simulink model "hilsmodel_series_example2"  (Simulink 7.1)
settings: Solver=ode3  StartTime=0.0  StopTime=1800  FixedStep=hilsmdl.simulation.stepsize.value  MaxStep=0.01  RelTol=1e-3  AbsTol=1e-3
undefined symbols (not defined in the file or in its folder): hilsmdl
libraries: HILS_model_library x9, simulink_extras x1

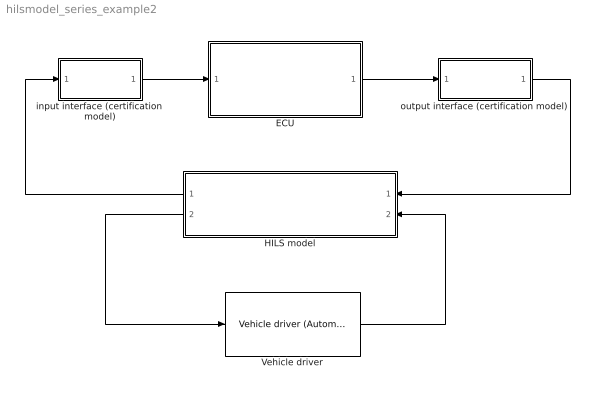
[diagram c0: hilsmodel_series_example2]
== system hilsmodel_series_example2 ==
  ECU : Subsystem  mask{dat=hilsmdl.ecu}
      mask prompts: dat "Data set for ECU"
  HILS model : Subsystem  Orientation=left
  Vehicle driver : HILS_model_library/Driver/Vehicle driver (Automatic)  dat=hilsmdl.driverautomatic
  input interface (certification model) : Subsystem
  output interface (certification model) : Subsystem
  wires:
  input interface (certification model)/1(to ECU) -> ECU/1(sensor in)
  ECU/1(cmd out) -> output interface (certification model)/1(from ECU)
  HILS model/1(To Ctrl) -> input interface (certification model)/1(plant in)
  output interface (certification model)/1(cmd out) -> HILS model/1(From Ctrl)
  Vehicle driver/1 -> HILS model/2(From driver)
  HILS model/2(To driver) -> Vehicle driver/1

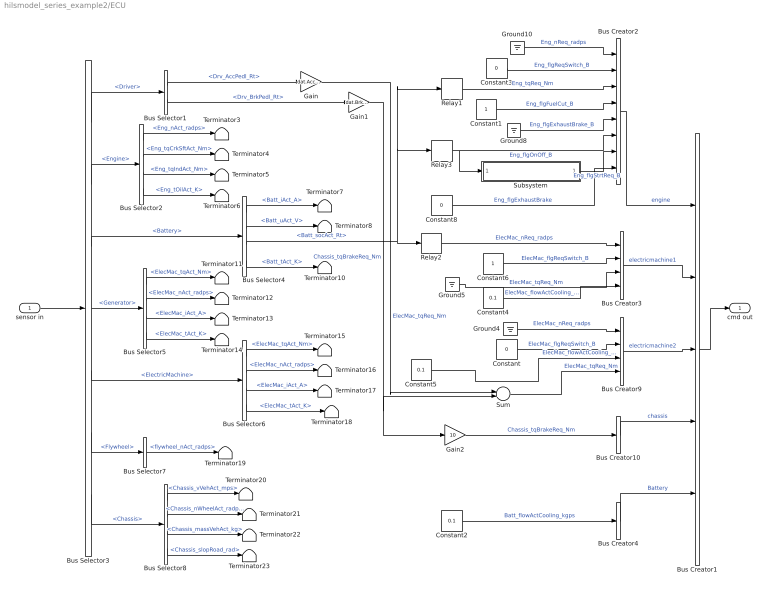
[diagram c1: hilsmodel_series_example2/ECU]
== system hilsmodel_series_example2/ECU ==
  sensor in : Inport
  Bus Creator1 : BusCreator  Inputs=5
  Bus Creator10 : BusCreator  Inputs=1
  Bus Creator2 : BusCreator  Inputs=8
  Bus Creator3 : BusCreator
  Bus Creator4 : BusCreator  Inputs=1
  Bus Creator9 : BusCreator
  Bus Selector1 : BusSelector  OutputSignals=Drv_AccPedl_Rt,Drv_BrkPedl_Rt
  Bus Selector2 : BusSelector  OutputSignals=Eng_nAct_radps,Eng_tqCrkSftAct_Nm,Eng_tqIndAct_Nm,Eng_tOilAct_K
  Bus Selector3 : BusSelector  OutputSignals=Driver,Engine,Battery,Generator,ElectricMachine,Flywheel,Chassis
  Bus Selector4 : BusSelector  OutputSignals=Batt_iAct_A,Batt_uAct_V,Batt_socAct_Rt,Batt_tAct_K
  Bus Selector5 : BusSelector  OutputSignals=ElecMac_tqAct_Nm,ElecMac_nAct_radps,ElecMac_iAct_A,ElecMac_tAct_K
  Bus Selector6 : BusSelector  OutputSignals=ElecMac_tqAct_Nm,ElecMac_nAct_radps,ElecMac_iAct_A,ElecMac_tAct_K
  Bus Selector7 : BusSelector  OutputSignals=flywheel_nAct_radps
  Bus Selector8 : BusSelector  OutputSignals=Chassis_vVehAct_mps,Chassis_nWheelAct_radps,Chassis_massVehAct_kg,Chassis_slopRoad_rad
  Constant : Constant  Value=0
  Constant1 : Constant
  Constant2 : Constant  Value=0.1
  Constant3 : Constant  Value=0
  Constant4 : Constant  Value=0.1
  Constant5 : Constant  Value=0.1
  Constant6 : Constant
  Constant8 : Constant  Value=0
  Gain : Gain  Gain=dat.AccPedalGain.value
  Gain1 : Gain  Gain=dat.BrkPedalGain.value
  Gain2 : Gain  Gain=10
  Ground{4..5,8,10} (4 alike) : Ground
  Relay1 : Relay  OnSwitchValue=dat.socstrategy.EngineOff.value  OffSwitchValue=dat.socstrategy.EngineOn.value  OnOutputValue=0  OffOutputValue=dat.socstrategy.torqueref.value
  Relay2 : Relay  OnSwitchValue=dat.socstrategy.EngineOff.value  OffSwitchValue=dat.socstrategy.EngineOn.value  OnOutputValue=0  OffOutputValue=dat.socstrategy.speedref.value
  Relay3 : Relay  OnSwitchValue=dat.socstrategy.EngineOff.value  OffSwitchValue=dat.socstrategy.EngineOn.value  OnOutputValue=0  OffOutputValue=1
  Subsystem : Subsystem
  Sum : Sum  Inputs=|+-
  Terminator{3..8,10..23} (20 alike) : Terminator
  cmd out : Outport
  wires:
  Bus Creator10/1 -> Bus Creator1/4  "chassis"
  Constant/1 -> Bus Creator9/2  "ElecMac_flgReqSwitch_B"
  Ground4/1 -> Bus Creator9/1  "ElecMac_nReq_radps"
  Bus Creator1/1 -> cmd out/1
  Bus Creator2/1 -> Bus Creator1/1  "engine"
  Ground10/1 -> Bus Creator2/1  "Eng_nReq_radps"
  Constant3/1 -> Bus Creator2/2  "Eng_flgReqSwitch_B"
  Bus Creator3/1 -> Bus Creator1/2  "electricmachine1"
  Constant6/1 -> Bus Creator3/2  "ElecMac_flgReqSwitch_B"
  Ground5/1 -> Bus Creator3/3  "ElecMac_tqReq_Nm"
  Bus Creator9/1 -> Bus Creator1/3  "electricmachine2"
  Bus Selector3/4 -> Bus Selector5/1  "<Generator>"
  sensor in/1 -> Bus Selector3/1
  Bus Selector3/1 -> Bus Selector1/1  "<Driver>"
  Bus Selector3/2 -> Bus Selector2/1  "<Engine>"
  Bus Selector3/3 -> Bus Selector4/1  "<Battery>"
  Bus Selector3/5 -> Bus Selector6/1  "<ElectricMachine>"
  Bus Selector3/6 -> Bus Selector7/1  "<Flywheel>"
  Bus Selector3/7 -> Bus Selector8/1  "<Chassis>"
  Bus Selector1/1 -> Gain/1  "<Drv_AccPedl_Rt>"
  Bus Selector1/2 -> Gain1/1  "<Drv_BrkPedl_Rt>"
  Bus Selector2/1 -> Terminator3/1  "<Eng_nAct_radps>"
  Bus Selector2/2 -> Terminator4/1  "<Eng_tqCrkSftAct_Nm>"
  Bus Selector2/3 -> Terminator5/1  "<Eng_tqIndAct_Nm>"
  Bus Selector2/4 -> Terminator6/1  "<Eng_tOilAct_K>"
  Bus Selector4/1 -> Terminator7/1  "<Batt_iAct_A>"
  Bus Selector4/2 -> Terminator8/1  "<Batt_uAct_V>"
  Bus Selector4/3 -> Relay2/1, Relay1/1, Relay3/1  "<Batt_socAct_Rt>"
  Bus Selector4/4 -> Terminator10/1  "<Batt_tAct_K>"
  Bus Selector5/1 -> Terminator11/1  "<ElecMac_tqAct_Nm>"
  Bus Selector5/2 -> Terminator12/1  "<ElecMac_nAct_radps>"
  Bus Selector5/3 -> Terminator13/1  "<ElecMac_iAct_A>"
  Bus Selector5/4 -> Terminator14/1  "<ElecMac_tAct_K>"
  Bus Selector6/1 -> Terminator15/1  "<ElecMac_tqAct_Nm>"
  Bus Selector6/2 -> Terminator16/1  "<ElecMac_nAct_radps>"
  Bus Selector6/3 -> Terminator17/1  "<ElecMac_iAct_A>"
  Bus Selector6/4 -> Terminator18/1  "<ElecMac_tAct_K>"
  Bus Selector7/1 -> Terminator19/1  "<flywheel_nAct_radps>"
  Bus Selector8/1 -> Terminator20/1  "<Chassis_vVehAct_mps>"
  Bus Selector8/2 -> Terminator21/1  "<Chassis_nWheelAct_radps>"
  Bus Selector8/3 -> Terminator22/1  "<Chassis_massVehAct_kg>"
  Bus Selector8/4 -> Terminator23/1  "<Chassis_slopRoad_rad>"
  Gain/1 -> Sum/1  "ElecMac_tqReq_Nm"
  Sum/1 -> Bus Creator9/4  "ElecMac_tqReq_Nm"
  Gain1/1 -> Gain2/1, Sum/2  "Chassis_tqBrakeReq_Nm"
  Relay1/1 -> Bus Creator2/3  "Eng_tqReq_Nm"
  Relay2/1 -> Bus Creator3/1  "ElecMac_nReq_radps"
  Ground8/1 -> Bus Creator2/5  "Eng_flgExhaustBrake_B"
  Constant1/1 -> Bus Creator2/4  "Eng_flgFuelCut_B"
  Relay3/1 -> Bus Creator2/6, Subsystem/1(Engine onoff)  "Eng_flgOnOff_B"
  Subsystem/1(Starter motor ctrl) -> Bus Creator2/7  "Eng_flgStrtReq_B"
  Bus Creator4/1 -> Bus Creator1/5  "Battery"
  Constant2/1 -> Bus Creator4/1  "Batt_flowActCooling_kgps"
  Constant4/1 -> Bus Creator3/4  "ElecMac_flowActCooling_kgps"
  Constant5/1 -> Bus Creator9/3  "ElecMac_flowActCooling_kgps"
  Constant8/1 -> Bus Creator2/8  "Eng_flgExhaustBrake"
  Gain2/1 -> Bus Creator10/1  "Chassis_tqBrakeReq_Nm"

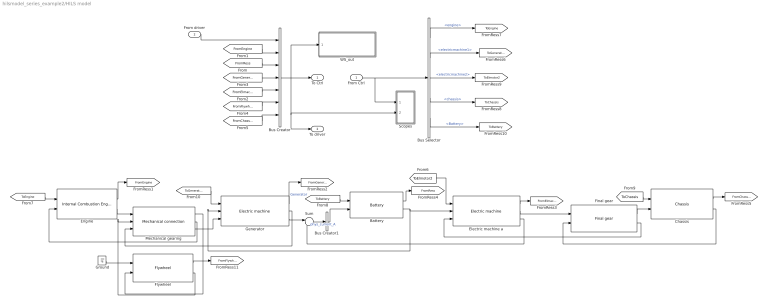
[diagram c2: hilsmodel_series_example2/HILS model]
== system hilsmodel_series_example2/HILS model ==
  From Ctrl : Inport
  From driver : Inport  Port=2
  Battery : HILS_model_library/Rechargable energy storage systems/Battery  dat=hilsmdl.battery
  Bus Creator : BusCreator  Inputs=7
  Bus Creator1 : BusCreator  Inputs=1
  Bus Selector : BusSelector  OutputSignals=engine,electricmachine1,electricmachine2,chassis,Battery
  Chassis : HILS_model_library/Chassis/Chassis  dat=hilsmdl.chassis
  Electric machine a : HILS_model_library/Energy converters/Electric machine  dat=hilsmdl.elmachinea
  Engine : HILS_model_library/Energy converters/Internal Combustion Engine  dat=hilsmdl.eng
  Final gear : HILS_model_library/Mechanical components/Final gear  dat=hilsmdl.finalgear
  Flywheel : HILS_model_library/Rechargable energy storage systems/Flywheel  dat=hilsmdl.flywheel
  Generator : HILS_model_library/Energy converters/Electric machine  dat=hilsmdl.elmachineb
  Ground : Ground
  Mechanical gearing : HILS_model_library/Mechanical components/Mechanical connection  dat=hilsmdl.mechconnection
  Scopes : Subsystem
  Sum : Sum  Inputs=|++
  WS_out : Subsystem
  To Ctrl : Outport
  To driver : Outport  Port=2
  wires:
  Bus Creator/1 -> To Ctrl/1, WS_out/1(from model), Scopes/2(plnt in), To driver/1
  From driver/1 -> Bus Creator/1
  Chassis/1 -> [FromChassis]
  From Ctrl/1 -> Scopes/1(ctrl in), Bus Selector/1
  [FromRess] -> Bus Creator/3
  Engine/1 -> [FromEngine]
  [FromEngine] -> Bus Creator/2
  [FromElmachine2] -> Bus Creator/5
  [FromGenerator1] -> Bus Creator/4
  [FromFlywheel] -> Bus Creator/6
  [FromChassis] -> Bus Creator/7
  Bus Selector/1 -> [ToEngine]  "<engine>"
  Bus Selector/2 -> [ToGenerator1]  "<electricmachine1>"
  [ToEngine] -> Engine/1
  [ToChassis] -> Chassis/1
  Electric machine a/1 -> [FromElmachine2]
  [ToElmotor2] -> Electric machine a/1
  Electric machine a/3 -> Sum/2
  Battery/2 -> Electric machine a/2, Generator/2
  Battery/1 -> [FromRess]
  [ToBattery] -> Battery/1
  Mechanical gearing/1 -> Flywheel/2
  Generator/2 -> Mechanical gearing/3
  Mechanical gearing/2 -> Engine/2
  Mechanical gearing/3 -> Generator/3
  Generator/1 -> [FromGenerator1]  "Generator"
  [ToGenerator1] -> Generator/1
  Flywheel/2 -> Mechanical gearing/2
  Flywheel/1 -> [FromFlywheel]
  Ground/1 -> Flywheel/1
  Bus Selector/4 -> [ToChassis]  "<chassis>"
  Bus Selector/3 -> [ToElmotor2]  "<electricmachine2>"
  Sum/1 -> Bus Creator1/1  "phys_current_A"
  Bus Creator1/1 -> Battery/2
  Engine/2 -> Mechanical gearing/1
  Generator/3 -> Sum/1
  Electric machine a/2 -> Final gear/1
  Final gear/2 -> Electric machine a/3
  Final gear/1 -> Chassis/2
  Chassis/2 -> Final gear/2
  Bus Selector/5 -> [ToBattery]  "<Battery>"

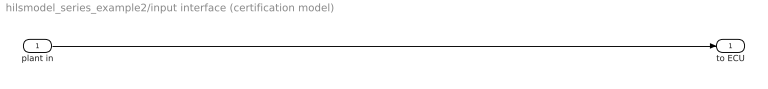
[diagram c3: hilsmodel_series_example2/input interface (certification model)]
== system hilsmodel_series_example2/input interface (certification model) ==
  plant in : Inport
  to ECU : Outport
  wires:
  plant in/1 -> to ECU/1

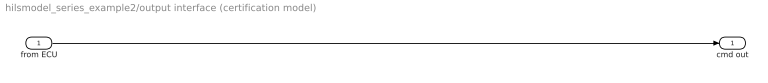
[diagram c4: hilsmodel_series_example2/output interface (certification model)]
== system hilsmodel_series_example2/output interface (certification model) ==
  from ECU : Inport
  cmd out : Outport
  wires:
  from ECU/1 -> cmd out/1

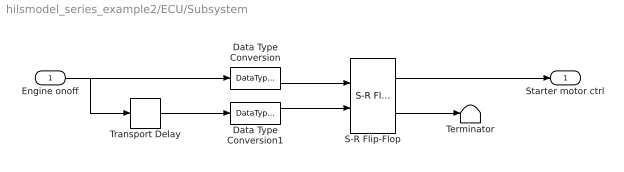
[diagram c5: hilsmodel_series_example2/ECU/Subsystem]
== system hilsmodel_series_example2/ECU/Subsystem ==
  Engine onoff : Inport
  Data Type Conversion : DataTypeConversion
  Data Type Conversion1 : DataTypeConversion
  S-R Flip-Flop : simulink_extras/Flip Flops/S-R Flip-Flop  initial_condition=0
  Terminator : Terminator
  Transport Delay : TransportDelay  DelayTime=dat.crankingtime.value
  Starter motor ctrl : Outport
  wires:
  Engine onoff/1 -> Transport Delay/1, Data Type Conversion/1
  S-R Flip-Flop/1 -> Starter motor ctrl/1
  S-R Flip-Flop/2 -> Terminator/1
  Transport Delay/1 -> Data Type Conversion1/1
  Data Type Conversion/1 -> S-R Flip-Flop/1
  Data Type Conversion1/1 -> S-R Flip-Flop/2

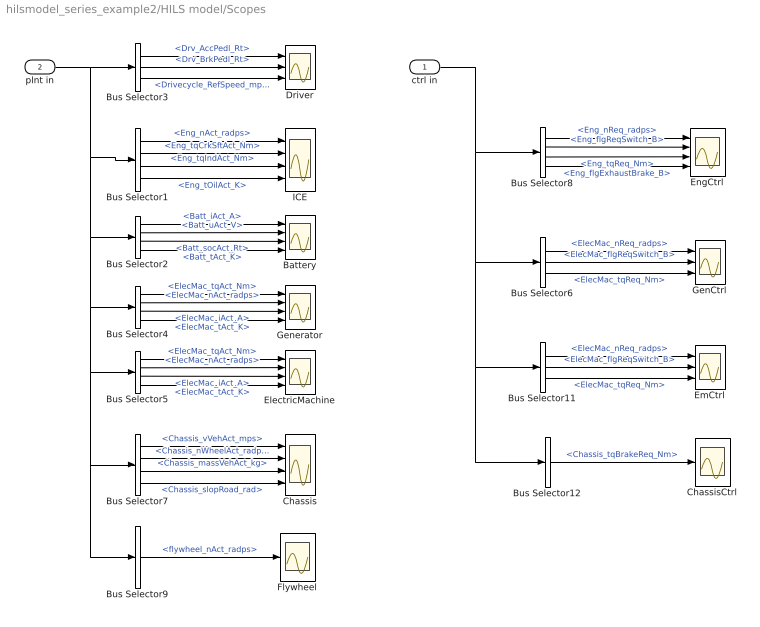
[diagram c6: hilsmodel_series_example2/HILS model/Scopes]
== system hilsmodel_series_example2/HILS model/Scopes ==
  ctrl in : Inport
  plnt in : Inport  Port=2
  Battery : Scope  NumInputPorts=4
  Bus Selector1 : BusSelector  OutputSignals=Engine.Eng_nAct_radps,Engine.Eng_tqCrkSftAct_Nm,Engine.Eng_tqIndAct_Nm,Engine.Eng_tOilAct_K
  Bus Selector11 : BusSelector  OutputSignals=electricmachine2.ElecMac_nReq_radps,electricmachine2.ElecMac_flgReqSwitch_B,electricmachine2.ElecMac_tqReq_Nm
  Bus Selector12 : BusSelector  OutputSignals=chassis.Chassis_tqBrakeReq_Nm
  Bus Selector2 : BusSelector  OutputSignals=Battery.Batt_iAct_A,Battery.Batt_uAct_V,Battery.Batt_socAct_Rt,Battery.Batt_tAct_K
  Bus Selector3 : BusSelector  OutputSignals=Driver.Drv_AccPedl_Rt,Driver.Drv_BrkPedl_Rt,Driver.Drivecycle_RefSpeed_mps
  Bus Selector4 : BusSelector  OutputSignals=Generator.ElecMac_tqAct_Nm,Generator.ElecMac_nAct_radps,Generator.ElecMac_iAct_A,Generator.ElecMac_tAct_K
  Bus Selector5 : BusSelector  OutputSignals=ElectricMachine.ElecMac_tqAct_Nm,ElectricMachine.ElecMac_nAct_radps,ElectricMachine.ElecMac_iAct_A,ElectricMachine.ElecMac_tAct_K
  Bus Selector6 : BusSelector  OutputSignals=electricmachine1.ElecMac_nReq_radps,electricmachine1.ElecMac_flgReqSwitch_B,electricmachine1.ElecMac_tqReq_Nm
  Bus Selector7 : BusSelector  OutputSignals=Chassis.Chassis_vVehAct_mps,Chassis.Chassis_nWheelAct_radps,Chassis.Chassis_massVehAct_kg,Chassis.Chassis_slopRoad_rad
  Bus Selector8 : BusSelector  OutputSignals=engine.Eng_nReq_radps,engine.Eng_flgReqSwitch_B,engine.Eng_tqReq_Nm,engine.Eng_flgExhaustBrake_B
  Bus Selector9 : BusSelector  OutputSignals=Flywheel.flywheel_nAct_radps
  Chassis : Scope  NumInputPorts=4
  ChassisCtrl : Scope
  Driver : Scope  NumInputPorts=3
  ElectricMachine : Scope  NumInputPorts=4
  EmCtrl : Scope  NumInputPorts=3
  EngCtrl : Scope  NumInputPorts=4
  Flywheel : Scope
  GenCtrl : Scope  NumInputPorts=3
  Generator : Scope  NumInputPorts=4
  ICE : Scope  NumInputPorts=4
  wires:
  Bus Selector3/1 -> Driver/1  "<Drv_AccPedl_Rt>"
  Bus Selector3/3 -> Driver/3  "<Drivecycle_RefSpeed_mps>"
  Bus Selector3/2 -> Driver/2  "<Drv_BrkPedl_Rt>"
  plnt in/1 -> Bus Selector3/1, Bus Selector1/1, Bus Selector2/1, Bus Selector5/1, Bus Selector7/1, Bus Selector9/1, Bus Selector4/1
  Bus Selector1/1 -> ICE/1  "<Eng_nAct_radps>"
  Bus Selector1/2 -> ICE/2  "<Eng_tqCrkSftAct_Nm>"
  Bus Selector1/3 -> ICE/3  "<Eng_tqIndAct_Nm>"
  Bus Selector2/1 -> Battery/1  "<Batt_iAct_A>"
  Bus Selector2/2 -> Battery/2  "<Batt_uAct_V>"
  Bus Selector2/3 -> Battery/3  "<Batt_socAct_Rt>"
  Bus Selector5/1 -> ElectricMachine/1  "<ElecMac_tqAct_Nm>"
  Bus Selector5/2 -> ElectricMachine/2  "<ElecMac_nAct_radps>"
  Bus Selector7/1 -> Chassis/1  "<Chassis_vVehAct_mps>"
  Bus Selector7/2 -> Chassis/2  "<Chassis_nWheelAct_radps>"
  Bus Selector7/3 -> Chassis/3  "<Chassis_massVehAct_kg>"
  Bus Selector7/4 -> Chassis/4  "<Chassis_slopRoad_rad>"
  ctrl in/1 -> Bus Selector8/1, Bus Selector11/1, Bus Selector12/1, Bus Selector6/1
  Bus Selector8/1 -> EngCtrl/1  "<Eng_nReq_radps>"
  Bus Selector8/2 -> EngCtrl/2  "<Eng_flgReqSwitch_B>"
  Bus Selector11/1 -> EmCtrl/1  "<ElecMac_nReq_radps>"
  Bus Selector11/2 -> EmCtrl/2  "<ElecMac_flgReqSwitch_B>"
  Bus Selector11/3 -> EmCtrl/3  "<ElecMac_tqReq_Nm>"
  Bus Selector12/1 -> ChassisCtrl/1  "<Chassis_tqBrakeReq_Nm>"
  Bus Selector1/4 -> ICE/4  "<Eng_tOilAct_K>"
  Bus Selector2/4 -> Battery/4  "<Batt_tAct_K>"
  Bus Selector4/1 -> Generator/1  "<ElecMac_tqAct_Nm>"
  Bus Selector4/2 -> Generator/2  "<ElecMac_nAct_radps>"
  Bus Selector4/3 -> Generator/3  "<ElecMac_iAct_A>"
  Bus Selector4/4 -> Generator/4  "<ElecMac_tAct_K>"
  Bus Selector5/3 -> ElectricMachine/3  "<ElecMac_iAct_A>"
  Bus Selector5/4 -> ElectricMachine/4  "<ElecMac_tAct_K>"
  Bus Selector8/3 -> EngCtrl/3  "<Eng_tqReq_Nm>"
  Bus Selector8/4 -> EngCtrl/4  "<Eng_flgExhaustBrake_B>"
  Bus Selector6/1 -> GenCtrl/1  "<ElecMac_nReq_radps>"
  Bus Selector6/2 -> GenCtrl/2  "<ElecMac_flgReqSwitch_B>"
  Bus Selector6/3 -> GenCtrl/3  "<ElecMac_tqReq_Nm>"
  Bus Selector9/1 -> Flywheel/1  "<flywheel_nAct_radps>"

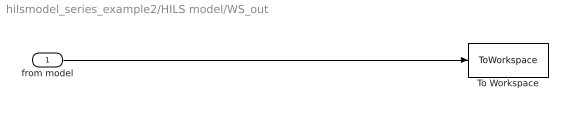
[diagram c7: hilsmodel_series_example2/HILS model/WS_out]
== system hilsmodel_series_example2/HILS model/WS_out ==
  from model : Inport
  To Workspace : ToWorkspace  VariableName=certmdl_out  SampleTime=hilsmdl.simulation.sampletime.value  SaveFormat=Structure With Time
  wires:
  from model/1 -> To Workspace/1
